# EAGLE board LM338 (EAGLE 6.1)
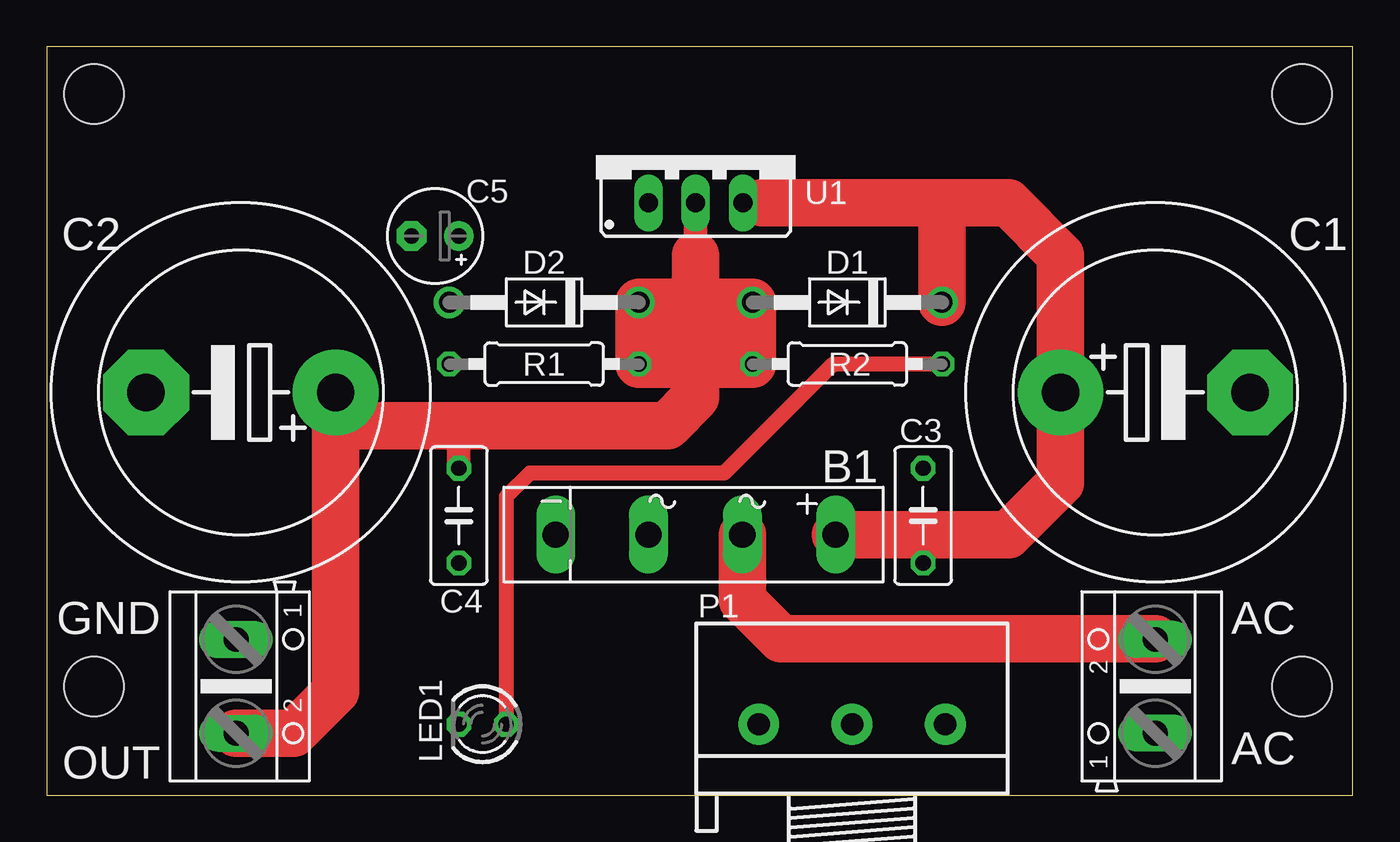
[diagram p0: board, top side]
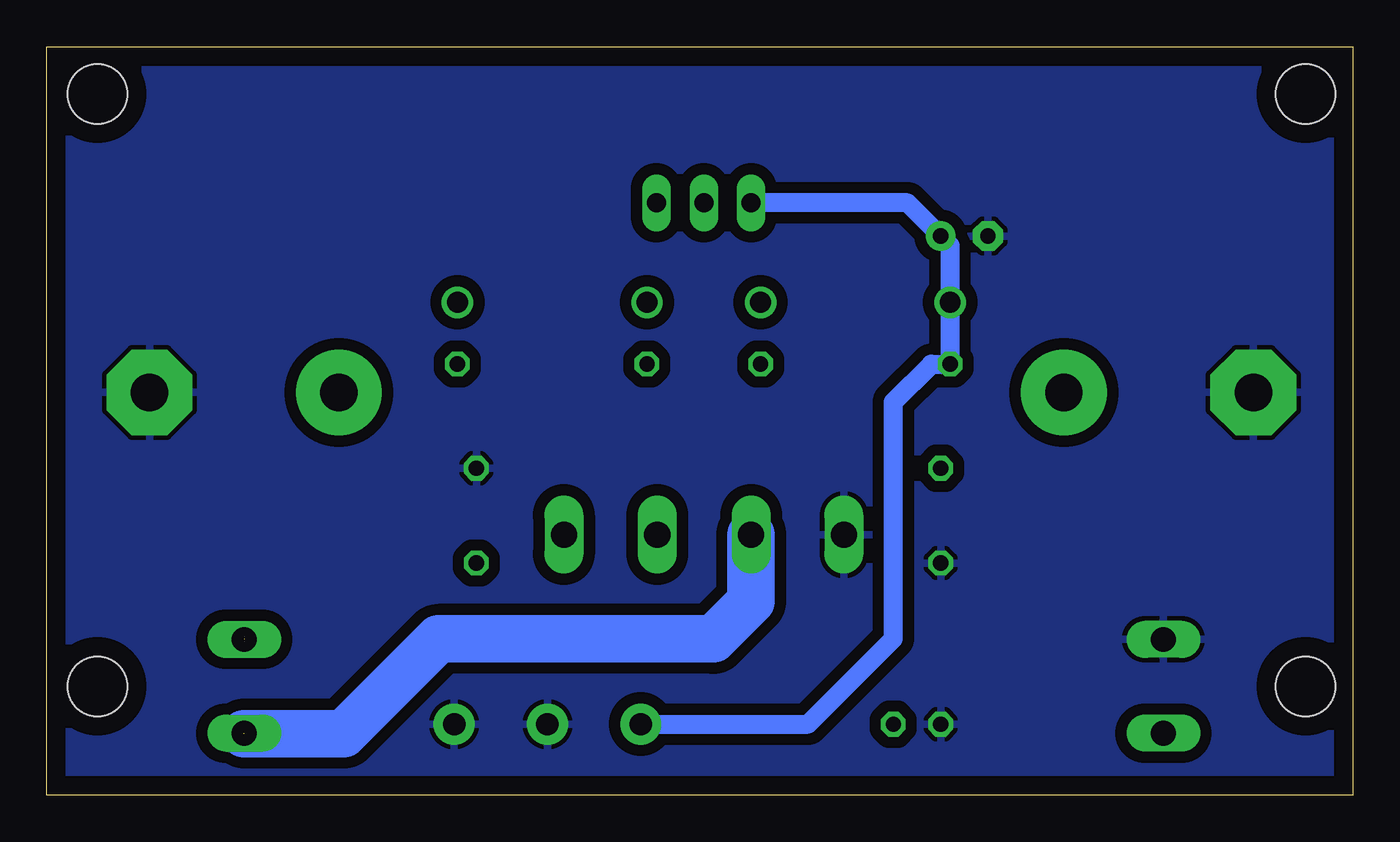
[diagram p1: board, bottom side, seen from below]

Size 70.03 x 40.12 mm. Coordinates in mm from the lower left corner, seen from the top.
Outline: 0,0 70.03,0 70.03,40.12 0,40.12 0,0
Copper layers (1*16): Top 0.035mm / dielectric 1.5mm / Bottom 0.035mm
Design rules: minimum track width 10mil, minimum drill 24mil, track to track 8mil, track to pad 8mil, pad to pad 8mil, via to via 8mil, smd to smd 8mil, copper to edge 40mil, drill to drill 8mil, minimum pad ring 10mil, minimum via ring 8mil, stop-mask expansion 4mil, vias tented up to drill 0mil, thermal gap 10mil
Holes 3.2 mm at 2.54,5.84 67.31,5.84 67.31,37.59 2.54,37.59

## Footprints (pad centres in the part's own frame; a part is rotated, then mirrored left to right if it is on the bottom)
AK500/2 = drill 1.321 long: 1 -2.515,0; 2 2.515,0
FB15 = drill 1.4 long: + -7.5,0; - 7.511,0; AC1 -2.496,0; AC2 2.533,0
EB20D = drill 2.007 pad 4.597: + -5.08,0 | drill 2.007 pad 4.597 octagon: - 5.08,0
C050-030X075 = drill 0.813 octagon: 1 -2.54,0; 2 2.54,0
E2,5-5 = drill 0.813 pad 1.6: + -1.27,0 | drill 0.813 pad 1.6 octagon: - 1.27,0
DO41-10 = drill 1.118: A 5.08,0; C -5.08,0
LED3MM = drill 0.813 octagon: A -1.27,0; K 1.27,0
3RP/1610N = drill 1.2 pad 2.184: 1 -5,0; 2 0,0; 3 5,0
0207/10 = drill 0.813 octagon: 1 -5.08,0; 2 5.08,0
TO220S = drill 1.016 long: 1 -2.54,-2.54; 2 0,-2.54; 3 2.54,-2.54

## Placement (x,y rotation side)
AC  [AK500/2]  59.44,5.84 90 top
B1  [FB15]  34.8,13.97 180 top
C1  4700uF  [EB20D]  59.44,21.59 0 top
C2  4700uF  [EB20D]  10.41,21.59 180 top
C3  100nF  [C050-030X075]  46.99,14.99 90 top
C4  100nF  [C050-030X075]  22.1,14.99 270 top
C5  10u  [E2,5-5]  20.83,29.97 180 top
D1  1N4007  [DO41-10]  42.93,26.42 180 top
D2  1N4007  [DO41-10]  26.67,26.42 180 top
LED1  [LED3MM]  23.37,3.81 180 top
OUT  [AK500/2]  10.16,5.84 270 top
P1  10k  [3RP/1610N]  43.18,3.81 0 top
R1  300  [0207/10]  26.67,23.11 0 top
R2  2,2k  [0207/10]  42.93,23.11 180 top
U1  LM338  [TO220S]  34.8,34.29 0 top

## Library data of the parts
AC OUT = con-ptr500; OC_FARNELL: unknown; OC_NEWARK: unknown
B1 = rectifier
C1-C5 R1 R2 = rcl
D1 D2 = diode
LED1 = led
P1 = pot
U1 = v-reg-3

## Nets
GND: B1.- C1.- C2.- C3.2 C4.2 C5.- LED1.K OUT.1 P1.2 P1.3
N$1: AC.2 B1.AC1
N$2: AC.1 B1.AC2
N$3: B1.+ C1.+ C3.1 D1.C U1.3
N$5: LED1.A R2.1
N$6: C2.+ C4.1 D1.A D2.C OUT.2 R1.2 R2.2 U1.2
N$7: C5.+ D2.A P1.1 R1.1 U1.1

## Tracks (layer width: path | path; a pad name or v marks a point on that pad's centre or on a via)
GND
  pour Bottom (isolate 0.61): 0,40.39 70.1,40.39 70.1,0 0,0
N$1  (1 unrouted)
  Top 2.54: B1.AC1 37.29,10.46 39.37,8.38 59.44,8.38
N$2  (1 unrouted)
  Bottom 2.54: B1.AC2 32.27,10.41 34.29,8.38 49.02,8.38 54.1,3.3 59.44,3.3
N$3
  Top 1.27: C3.1 46.99,13.97 | 38.35,31.75 U1.3
  Top 2.54: B1.+ 46.99,13.97 51.56,13.97 54.36,16.76 C1.+ 54.36,28.96 51.56,31.75 48.01,31.75 | 48.01,31.75 38.35,31.75 | D1.C 48.01,31.75
N$5
  Top 0.813: R2.1 42.16,23.11 36.32,17.27 25.91,17.27 24.64,16 LED1.A
N$6
  Top 1.27: U1.2 34.8,28.96 | C4.1 22.1,19.05 22.35,19.81
  Top 2.54: 34.8,26.42 34.8,21.34 33.27,19.81 22.35,19.81 15.47,19.81 15.47,21.57 C2.+ 15.49,5.59 13.23,3.33 OUT.2 | 34.8,26.42 34.8,28.96 | 34.8,26.42 D2.C R1.2 37.59,23.11 37.59,24.64 32.26,24.64 | 34.8,26.42 D1.A R2.2
N$7
  Bottom 1.016: U1.1 23.88,31.75 C5.+ 21.59,29.46 D2.A R1.1 22.61,23.11 24.64,21.08 24.64,8.38 29.21,3.81 P1.1

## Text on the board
tNames: GND | AC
